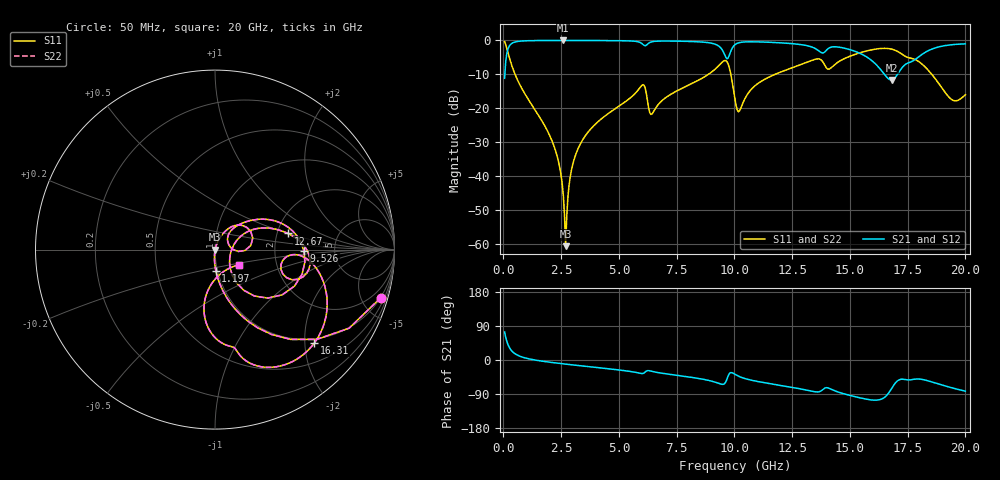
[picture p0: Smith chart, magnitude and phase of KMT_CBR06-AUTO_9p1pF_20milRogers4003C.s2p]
! Data measured by Modelithics Inc. support@modelithics.com 813-866-6335
! KEMET CBR06-AUTO 9.1pF, Pad Width= 0.851mm, Pad Length= 0.64mm, Pad Gap= 0.62mm, 20mil Rogers 4003C substrate Data, January 2022
# hz S ma R 50
! 2 Port Network Data from SP1.SP block
! freq  magS11  angS11  magS21  angS21  magS12  angS12  magS22  angS22
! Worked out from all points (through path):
!   401 points, 50 MHz to 20 GHz, reference 50 ohm
!   highest |S21| = -0.01 dB at 2.594 GHz (marker M1); lowest = -11.6 dB at 16.81 GHz (marker M2)
!   group delay of S21, straight-line fit = 13.1 ps
!   lowest |S11| = -60.6 dB at 2.693 GHz (marker M3), VSWR 1.00, Z = 50.1 - j0.0138 ohm
!   |S11| at or under -10 dB: 503.5 MHz to 8.87 GHz (8.366 GHz wide, 179 % of centre); 9.843 GHz to 11.76 GHz (1.913 GHz wide, 17.7 % of centre); 18.55 GHz to end of sweep
!   |S22| runs from -60.6 to -0.3 dB; largest |S21 - S12| = 0
!   S11 on the Smith chart (normalised r, x): 50 MHz: 0.98, -6.86; 1.197 GHz: 0.98, -0.23; 9.526 GHz: 2.97, -0.06; 12.67 GHz: 2.29, +0.50; 16.31 GHz: 0.90, -2.21; 20 GHz: 1.29, -0.22
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5e7  0.9609 -16.3  0.2767 73.7  0.2767 73.7  0.9609 -16.3
3.99125e8  0.3918 -68.5  0.9195 21.4  0.9195 21.4  0.3918 -68.5
1.197125e9  0.1167 -87.8  0.9924 1.9  0.9924 1.9  0.1167 -87.8
2.2445e9  0.02446 -95.7  0.9988 -7.7  0.9988 -7.7  0.02446 -95.7
2.593625e9  0.005149 -89.9  0.999 -10.2  0.999 -10.2  0.005149 -89.9
2.693375e9  0.0009355 -8.5  0.999 -10.9  0.999 -10.9  0.0009355 -8.5
2.992625e9  0.0146 73.2  0.9988 -12.9  0.9988 -12.9  0.0146 73.2
3.391625e9  0.03273 72.5  0.9983 -15.6  0.9983 -15.6  0.03273 72.5
5.985125e9  0.217 34.2  0.9045 -35.8  0.9045 -35.8  0.217 34.2
6.384125e9  0.08132 21.0  0.9458 -29.2  0.9458 -29.2  0.08132 21.0
6.73325e9  0.1171 48.7  0.9774 -33.6  0.9774 -33.6  0.1171 48.7
9.52625e9  0.496 -0.9  0.6723 -64.0  0.6723 -64.0  0.496 -0.9
1.0025e10  0.1363 -51.3  0.8666 -37.9  0.8666 -37.9  0.1363 -51.3
1.02245e10  0.09222 -1.1  0.9301 -44.0  0.9301 -44.0  0.09222 -1.1
1.266838e10  0.4157 12.5  0.8849 -74.1  0.8849 -74.1  0.4157 12.5
1.336662e10  0.5099 0.1  0.7968 -82.5  0.7968 -82.5  0.5099 0.1
1.630925e10  0.7596 -43.2  0.3796 -104.4  0.3796 -104.4  0.7596 -43.2
1.670825e10  0.755 -57.0  0.2667 -84.3  0.2667 -84.3  0.755 -57.0
1.6808e10  0.7437 -60.7  0.2617 -74.9  0.2617 -74.9  0.7437 -60.7
1.830425e10  0.3919 -98.0  0.681 -53.6  0.681 -53.6  0.3919 -98.0
1.94015e10  0.1352 -74.0  0.8641 -73.2  0.8641 -73.2  0.1352 -74.0
2e10  0.1586 -32.4  0.8897 -82.3  0.8897 -82.3  0.1586 -32.4
